DATA_BLOCK DB 75
TITLE =
VERSION : 0.0


  STRUCT
   MSigGrp : ARRAY  [1 .. 16 ] OF STRUCT
    MExtAdr : INT ;
    MFirstAdr : DINT ;
    MLastAdr : DINT ;
   END_STRUCT ;
  END_STRUCT ;
BEGIN
   MSigGrp[1].MExtAdr := 0;
   MSigGrp[1].MFirstAdr := L#0;
   MSigGrp[1].MLastAdr := L#0;
   MSigGrp[2].MExtAdr := 0;
   MSigGrp[2].MFirstAdr := L#0;
   MSigGrp[2].MLastAdr := L#0;
   MSigGrp[3].MExtAdr := 0;
   MSigGrp[3].MFirstAdr := L#0;
   MSigGrp[3].MLastAdr := L#0;
   MSigGrp[4].MExtAdr := 0;
   MSigGrp[4].MFirstAdr := L#0;
   MSigGrp[4].MLastAdr := L#0;
   MSigGrp[5].MExtAdr := 0;
   MSigGrp[5].MFirstAdr := L#0;
   MSigGrp[5].MLastAdr := L#0;
   MSigGrp[6].MExtAdr := 0;
   MSigGrp[6].MFirstAdr := L#0;
   MSigGrp[6].MLastAdr := L#0;
   MSigGrp[7].MExtAdr := 0;
   MSigGrp[7].MFirstAdr := L#0;
   MSigGrp[7].MLastAdr := L#0;
   MSigGrp[8].MExtAdr := 0;
   MSigGrp[8].MFirstAdr := L#0;
   MSigGrp[8].MLastAdr := L#0;
   MSigGrp[9].MExtAdr := 0;
   MSigGrp[9].MFirstAdr := L#0;
   MSigGrp[9].MLastAdr := L#0;
   MSigGrp[10].MExtAdr := 0;
   MSigGrp[10].MFirstAdr := L#0;
   MSigGrp[10].MLastAdr := L#0;
   MSigGrp[11].MExtAdr := 0;
   MSigGrp[11].MFirstAdr := L#0;
   MSigGrp[11].MLastAdr := L#0;
   MSigGrp[12].MExtAdr := 0;
   MSigGrp[12].MFirstAdr := L#0;
   MSigGrp[12].MLastAdr := L#0;
   MSigGrp[13].MExtAdr := 0;
   MSigGrp[13].MFirstAdr := L#0;
   MSigGrp[13].MLastAdr := L#0;
   MSigGrp[14].MExtAdr := 0;
   MSigGrp[14].MFirstAdr := L#0;
   MSigGrp[14].MLastAdr := L#0;
   MSigGrp[15].MExtAdr := 0;
   MSigGrp[15].MFirstAdr := L#0;
   MSigGrp[15].MLastAdr := L#0;
   MSigGrp[16].MExtAdr := 0;
   MSigGrp[16].MFirstAdr := L#0;
   MSigGrp[16].MLastAdr := L#0;
END_DATA_BLOCK

